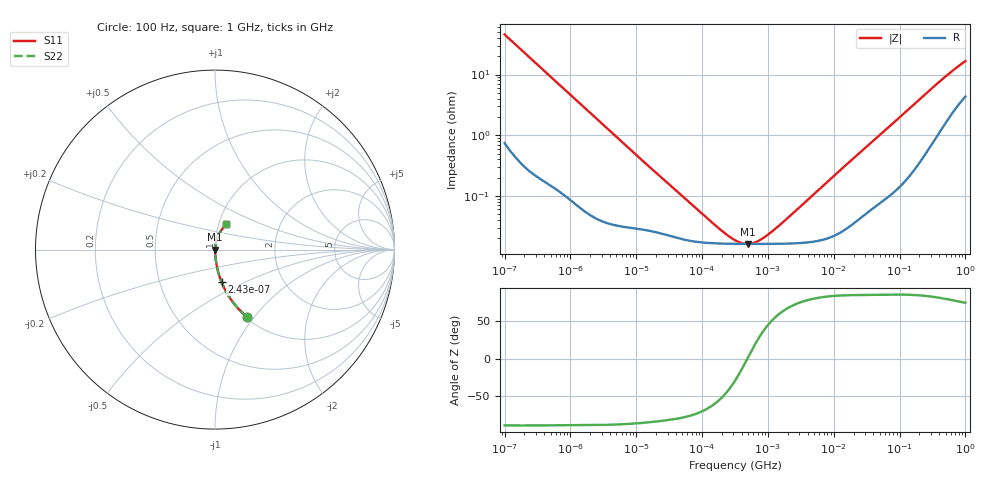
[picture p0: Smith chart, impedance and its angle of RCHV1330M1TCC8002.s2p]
! RCHV1330M1TCC8002  S-PARAMETER MODEL  (AEC-Q200 qualified)
! Model Generated by ELNA Corporation (http://www.ty-top.com)
! Version 1.0
! ELNA Control No. 240229
! Copyright (c) 2024 ELNA CO.,LTD. All Rights Reserved.
! Products Name : CONDUCTIVE POLYMER HYBRID ALUMINUM ELECTROLYTIC CAPACITORS
! Characteristics :
!  Capacitance  :  33uF  ,  Rated voltage  :  25V
!  Operating Temp. Range  :  -55 to +105 degC  ,  Endurance  :  5000hr at 105 degC
!  Dimension D  :  5mm  ,  Dimension L  :  5.8mm
! Frequency Range : 100Hz - 1GHz
! External Node Assignments :
!  1  o---| |---o  2
# MHz S RI R 50
!Freq[MHz].  S11 Real  S11 Imag  S21 Real  S21 Imag  S12 Real  S12 Imag  S22 Real  S22 Imag
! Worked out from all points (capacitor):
!   401 points, 100 Hz to 1 GHz, reference 50 ohm
!   read as one part in series: C = 34.8 uF near 108 Hz
!   lowest |Z| = 16.2 mohm at 492.6 kHz (marker M1)
!   series resonance near 486 kHz, so ESL is about 3.1 nH
!   S11 on the Smith chart (normalised r, x): 100 Hz: 1.01, -0.91; 243 Hz: 1.01, -0.38; 1 GHz: 1.09, +0.32
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0.0001  0.1766 -0.3733  0.8234 0.3733  0.8234 0.3733  0.1766 -0.3733
0.000113  0.1446 -0.3441  0.8554 0.3441  0.8554 0.3441  0.1446 -0.3441
0.000162  0.0766 -0.2593  0.9234 0.2593  0.9234 0.2593  0.0766 -0.2593
0.000243  0.0366 -0.1812  0.9634 0.1812  0.9634 0.1812  0.0366 -0.1812
0.000543  0.00849 -0.0839  0.9915 0.0839  0.9915 0.0839  0.00849 -0.0839
0.001488  0.00158 -0.0312  0.9984 0.0312  0.9984 0.0312  0.00158 -0.0312
0.004241  0.00046 -0.011  0.9995 0.011  0.9995 0.011  0.00046 -0.011
0.022131  0.000251 -0.00217  0.9997 0.00217  0.9997 0.00217  0.000251 -0.00217
0.165959  0.000166 -0.000268  0.9998 0.000268  0.9998 0.000268  0.000166 -0.000268
0.238506  0.000164 -0.00016  0.9998 0.00016  0.9998 0.00016  0.000164 -0.00016
0.316228  0.000163 -9.19e-05  0.9998 9.19e-05  0.9998 9.19e-05  0.000163 -9.19e-05
0.402717  0.000162 -3.92e-05  0.9998 3.92e-05  0.9998 3.92e-05  0.000162 -3.92e-05
0.492606  0.000162 2.84e-06  0.9998 -2.84e-06  0.9998 -2.84e-06  0.000162 2.84e-06
0.679986  0.000162 7.1e-05  0.9998 -7.1e-05  0.9998 -7.1e-05  0.000162 7.1e-05
0.977237  0.000162 0.000157  0.9998 -0.000157  0.9998 -0.000157  0.000162 0.000157
1.650061  0.000164 0.000322  0.9998 -0.000322  0.9998 -0.000322  0.000164 0.000322
4.704354  0.000176 0.000992  0.9998 -0.000992  0.9998 -0.000992  0.000176 0.000992
69.9842  0.00119 0.0139  0.9988 -0.0139  0.9988 -0.0139  0.00119 0.0139
184.0772  0.00434 0.0355  0.9957 -0.0355  0.9957 -0.0355  0.00434 0.0355
412.0975  0.0171 0.0748  0.9829 -0.0748  0.9829 -0.0748  0.0171 0.0748
695.825  0.0394 0.1136  0.9606 -0.1136  0.9606 -0.1136  0.0394 0.1136
1000  0.0637 0.1444  0.9363 -0.1444  0.9363 -0.1444  0.0637 0.1444
